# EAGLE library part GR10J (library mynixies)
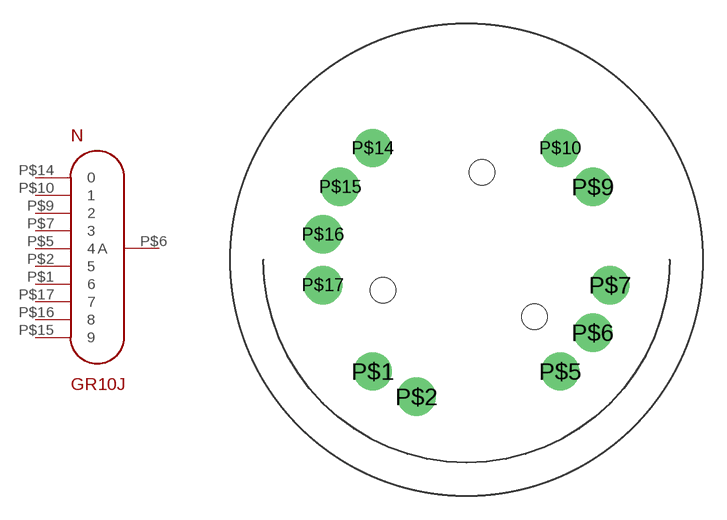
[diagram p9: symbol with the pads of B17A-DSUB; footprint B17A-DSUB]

Designator prefix N

## GR10JB17A  [B17A-DSUB]
P$1  6  pas
P$2  5  pas
P$5  4  pas
P$6  A  pas
P$7  3  pas
P$9  2  pas
P$10  1  pas
P$14  0  pas
P$15  9  pas
P$16  8  pas
P$17  7  pas

## Footprint B17A-DSUB (pad centres in mm)
drill 1.6: P$1 -5.861,-6.985; P$2 -3.119,-8.569; P$5 5.861,-6.985; P$6 7.897,-4.559; P$7 8.98,-1.583; P$9 7.897,4.559; P$10 5.861,6.985; P$14 -5.861,6.985; P$15 -7.897,4.559; P$16 -8.98,1.583; P$17 -8.98,-1.583
hole 1.6 at 0.964,5.466
hole 1.6 at -5.215,-1.898
hole 1.6 at 4.251,-3.567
